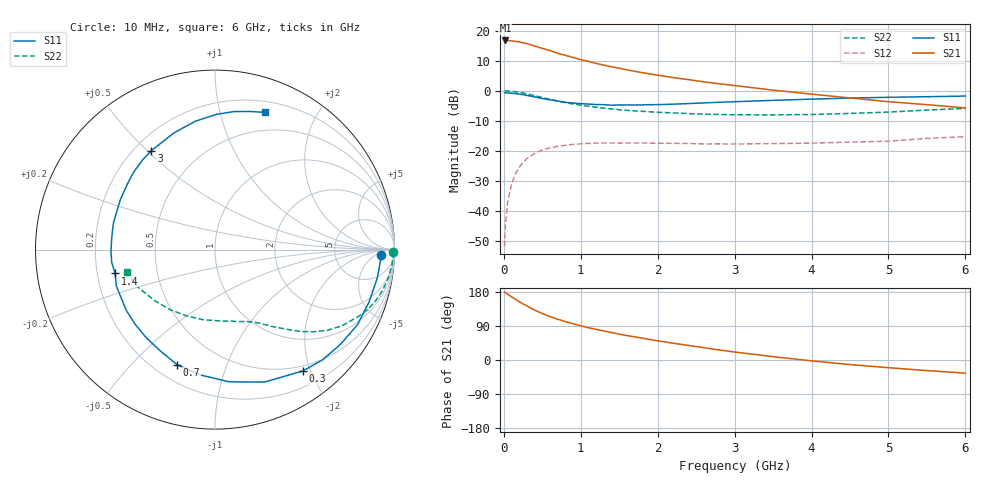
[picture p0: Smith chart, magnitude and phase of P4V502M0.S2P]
! SIEMENS Small Signal Semiconductors
! BFP182
! Si NPN RF Bipolar Junction Transistor in SOT143
! VCE = 0.5 V  IC = 2 mA
! Common Emitter S-Parameters:  March  1996
# GHz  S  MA  R  50
!  f  S11  S21  S12  S22
! GHz  MAG  ANG  MAG  ANG  MAG  ANG  MAG  ANG
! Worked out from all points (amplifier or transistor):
!   36 points, 10 MHz to 6 GHz, reference 50 ohm
!   highest |S21| = 16.7 dB at 20 MHz (marker M1)
!   |S21| within 3 dB of that: start of sweep to 550.3 MHz
!   unconditionally stable (mu >= 1): 1.978 GHz to end of sweep
!   at 250 MHz: K = 0.14, MSG = 19.9 dB, |S12| = -23.8 dB
!   at 1.4 GHz: K = 0.74, MSG = 12.7 dB, |S12| = -17.4 dB
!   at 6 GHz: K = 1.26, MAG = 1.7 dB, |S12| = -15.3 dB
!   S11 on the Smith chart (normalised r, x): 10 MHz: 22, -9; 300 MHz: 0.42, -1.88; 700 MHz: 0.29, -0.68; 1.4 GHz: 0.28, -0.11; 3 GHz: 0.27, +0.52; 6 GHz: 0.31, +1.39
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0.01  0.9244 -1.9  6.825 179.0  0.0026 87.3  0.9934 -0.8
0.02  0.9241 -3.8  6.838 178.0  0.0058 83.7  0.9943 -1.8
0.05  0.9182 -9.8  6.82 173.4  0.0142 86.3  0.9903 -4.5
0.1  0.9066 -18.9  6.725 166.8  0.0279 78.6  0.9797 -8.9
0.2  0.8756 -37.1  6.458 153.9  0.0533 68.1  0.942 -17.3
0.25  0.8583 -45.7  6.256 147.9  0.0642 63.2  0.9156 -21.3
0.3  0.8346 -54.1  6.054 142.7  0.0745 58.8  0.8845 -24.7
0.4  0.7881 -69.5  5.539 131.8  0.0908 50.8  0.8278 -30.7
0.5  0.7408 -83.9  5.044 122.6  0.1035 43.5  0.7707 -35.7
0.6  0.7034 -96.4  4.648 114.7  0.1123 37.9  0.716 -39.7
0.7  0.6751 -108.2  4.201 107.7  0.1189 33.0  0.6709 -42.9
0.8  0.6413 -118.4  3.873 101.3  0.1237 28.9  0.6323 -45.6
0.9  0.6236 -127.6  3.559 95.7  0.1281 25.3  0.6013 -47.7
1.1  0.5992 -145.4  3.062 85.1  0.133 19.7  0.5505 -51.8
1.4  0.5723 -166.6  2.499 72.5  0.1351 13.0  0.4972 -57.0
1.8  0.5803 170.3  1.997 57.5  0.1349 8.4  0.4539 -62.8
2.2  0.5965 152.0  1.65 44.3  0.1331 5.0  0.4268 -70.0
3  0.6557 122.7  1.218 21.1  0.13 2.5  0.3972 -87.0
3.5  0.6902 109.1  1.021 8.8  0.1319 2.4  0.3965 -99.2
4.5  0.7539 89.3  0.757 -12.1  0.1393 3.1  0.4186 -127.0
5.5  0.7936 75.9  0.585 -28.0  0.1609 3.6  0.4755 -153.4
6  0.8142 69.8  0.517 -34.7  0.1719 1.2  0.5079 -165.6
